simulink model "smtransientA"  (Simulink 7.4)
settings: Solver=ode45  StartTime=0.0  StopTime=5  MaxStep=1e-3  RelTol=1e-4  AbsTol=1e-4
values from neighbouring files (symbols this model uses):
  Bm = 0.10    (= 0.1)    [IMabc2.m]    (also in imabcparam.m = 0.01; IMabcrun0.m = 0.01; IMabcrun1.m = 0.001; IMcur0.m = 1e-06)
  H = 0.60    (= 0.6)    [IMabc2.m]    (also in IMcur0.m = 0.3; imdef0vec.m = 0.3; imdef1vec.m = 0.3; imdef2vec.m = 0.3)
  n0 = 0.98    [imdef0vec.m]    (also in imdef1vec.m = 0.978; imdef2vec.m; imdefrotflux.m; imdefSIvec1.m = 0.95)
  Ra = .95    (= 0.95)    [altwdgs.m]    (also in Ccurverun.m = 0.018)
  tc = abs(fco)    [im3phase.m]
  Te0 = 0.75/wo*p*(Is*conj(Is)*Req)    [imdefSIvec1.m]
  V = [Vas 0 0].'    [Actac.m]    (also in acttrcalc1.m = str2num(get(h,'string')); im3d.m = eval(get(hVs,'String')); IMabc2.m = [vas vbs vcs 0 0 0]'; IMabcf0.m = [vas vbs vcs 0 0 0]')
  wo = 2*pi*freq0    [calc0.m]    (also in IMabc2.m = 376.991118431; imabcparam.m = 376.991118431; IMabcrun0.m = 376.991118431; IMabcrun1.m = 376.991118431)
undefined symbols (not defined in the file or in its folder): delta0, fk0, L_1, phif0, Rf, Rkd, Rkq, vf0

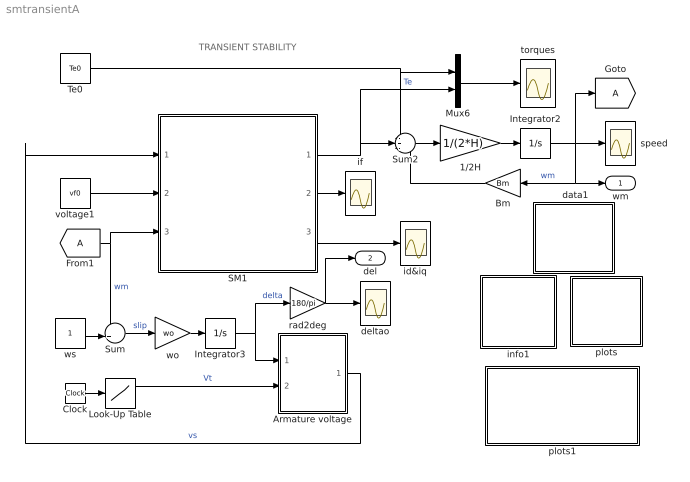
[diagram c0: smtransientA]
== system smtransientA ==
  note: TRANSIENT STABILITY
  " data1" : Subsystem
  1/2H : Gain  Gain=1/(2*H)  ParameterDataType=sfix(16)  ParameterScaling=2^0  OutDataType=sfix(16)  OutScaling=2^0
  Armature voltage : Subsystem
  Bm : Gain  Gain=Bm  ParameterDataType=sfix(16)  ParameterScaling=2^0  OutDataType=sfix(16)  OutScaling=2^0
  Clock : Clock
  Integrator2 : Integrator  InitialCondition=n0
  Integrator3 : Integrator  InitialCondition=delta0
  Look-Up Table : Lookup  InputValues=[0 0.5 0.5 0.5+tc 0.5+tc 3]  Table=[V V 0 0 V V]  OutDataType=sfix(16)  OutScaling=2^0
  Mux6 : Mux  Inputs=2
  SM1 : Subsystem
  Sum : Sum  Inputs=-+|  OutDataType=sfix(16)  OutScaling=2^0
  Sum2 : Sum  Inputs=-+-  OutDataType=sfix(16)  OutScaling=2^0
  Te0 : Constant  Value=Te0  OutDataType=sfix(16)  OutScaling=2^0
  deltao : Scope
  id&iq : Scope
  if : Scope
  info1 : Subsystem
  plots : Subsystem
  plots1 : Subsystem
  rad2deg : Gain  Gain=180/pi  ParameterDataType=sfix(16)  ParameterScaling=2^0  OutDataType=sfix(16)  OutScaling=2^0
  speed : Scope
  torques : Scope
  voltage1 : Constant  Value=vf0  OutDataType=sfix(16)  OutScaling=2^0
  wo : Gain  Gain=wo  ParameterDataType=sfix(16)  ParameterScaling=2^0  OutDataType=sfix(16)  OutScaling=2^0
  ws : Constant  OutDataType=sfix(16)  OutScaling=2^0
  wm : Outport
  del : Outport  Port=2
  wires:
  Mux6/1 -> torques/1
  voltage1/1 -> SM1/2(vf)
  SM1/2(if) -> if/1
  Sum2/1 -> 1/2H/1
  1/2H/1 -> Integrator2/1
  SM1/1(Te) -> Sum2/2, Mux6/2  "Te"
  Bm/1 -> Sum2/3
  Integrator2/1 -> speed/1, [A], Bm/1, wm/1  "wm"
  Te0/1 -> Mux6/1, Sum2/1
  ws/1 -> Sum/2
  Sum/1 -> wo/1  "slip"
  wo/1 -> Integrator3/1
  Armature voltage/1(vs) -> SM1/1(vs)  "vs"
  Integrator3/1 -> Armature voltage/1(delta), rad2deg/1  "delta"
  SM1/3(ia) -> id&iq/1
  rad2deg/1 -> deltao/1, del/1
  Clock/1 -> Look-Up Table/1
  Look-Up Table/1 -> Armature voltage/2(Vt)  "Vt"
  [A] -> Sum/1, SM1/3(wm)  "wm"

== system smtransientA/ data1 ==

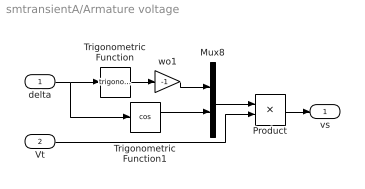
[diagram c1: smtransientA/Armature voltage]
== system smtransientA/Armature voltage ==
  delta : Inport  OutDataType=sfix(16)  OutScaling=2^0
  Vt : Inport  Port=2  OutDataType=sfix(16)  OutScaling=2^0
  Mux8 : Mux  Inputs=2
  Product : Product  OutDataType=sfix(16)  OutScaling=2^0
  Trigonometric Function : Trigonometry
  Trigonometric Function1 : Trigonometry  Operator=cos
  wo1 : Gain  Gain=-1  ParameterDataType=sfix(16)  ParameterScaling=2^0  OutDataType=sfix(16)  OutScaling=2^0
  vs : Outport
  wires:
  delta/1 -> Trigonometric Function/1, Trigonometric Function1/1
  Trigonometric Function/1 -> wo1/1
  Mux8/1 -> Product/1
  wo1/1 -> Mux8/1
  Trigonometric Function1/1 -> Mux8/2
  Product/1 -> vs/1
  Vt/1 -> Product/2

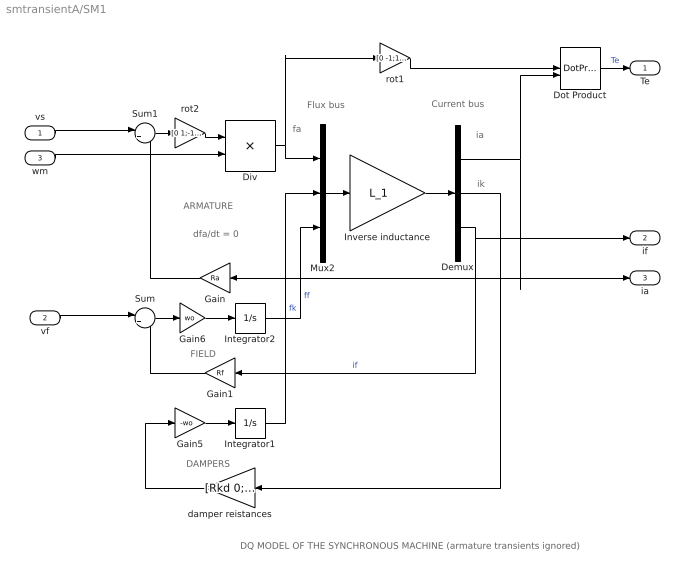
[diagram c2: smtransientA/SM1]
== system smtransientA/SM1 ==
  note: DAMPERS
  note: ARMATURE
  note: fa
  note: ia
  note: FIELD
  note: DQ MODEL OF THE SYNCHRONOUS MACHINE (armature transients ignored)
  note: Flux bus
  note: Current bus
  note: dfa/dt = 0
  note: ik
  vs : Inport  OutDataType=sfix(16)  OutScaling=2^0
  vf : Inport  Port=2  OutDataType=sfix(16)  OutScaling=2^0
  wm : Inport  Port=3  OutDataType=sfix(16)  OutScaling=2^0
  Demux : Demux  Outputs=3
  Div : Product  Inputs=*/  Multiplication=Matrix(*)  OutDataType=sfix(16)  OutScaling=2^0
  Dot Product : DotProduct  OutDataType=fixdt(1, 16)  OutScaling=2^-10
  Gain : Gain  Gain=Ra  ParameterDataType=sfix(16)  ParameterScaling=2^0  OutDataType=sfix(16)  OutScaling=2^0
  Gain1 : Gain  Gain=Rf  ParameterDataType=sfix(16)  ParameterScaling=2^0  OutDataType=sfix(16)  OutScaling=2^0
  Gain5 : Gain  Gain=-wo  ParameterDataType=sfix(16)  ParameterScaling=2^0  OutDataType=sfix(16)  OutScaling=2^0
  Gain6 : Gain  Gain=wo  ParameterDataType=sfix(16)  ParameterScaling=2^0  OutDataType=sfix(16)  OutScaling=2^0
  Integrator1 : Integrator  InitialCondition=fk0
  Integrator2 : Integrator  InitialCondition=phif0
  Inverse inductance : Gain  Gain=L_1  Multiplication=Matrix(K*u)  ParameterDataType=sfix(16)  ParameterScaling=2^0  OutDataType=sfix(16)  OutScaling=2^0
  Mux2 : Mux  Inputs=3
  Sum : Sum  Inputs=|+-  OutDataType=sfix(16)  OutScaling=2^0
  Sum1 : Sum  Inputs=|+-  OutDataType=sfix(16)  OutScaling=2^0
  damper reistances : Gain  Gain=[Rkd 0;0 Rkq]  Multiplication=Matrix(K*u)  ParameterDataType=sfix(16)  ParameterScaling=2^0  OutDataType=sfix(16)  OutScaling=2^0
  rot1 : Gain  Gain=[0 -1;1 0]  Multiplication=Matrix(K*u)  ParameterDataType=sfix(16)  ParameterScaling=2^0  OutDataType=sfix(16)  OutScaling=2^0
  rot2 : Gain  Gain=[0 1;-1 0]  Multiplication=Matrix(K*u)  ParameterDataType=sfix(16)  ParameterScaling=2^0  OutDataType=sfix(16)  OutScaling=2^0
  Te : Outport
  if : Outport  Port=2
  ia : Outport  Port=3
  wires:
  Gain5/1 -> Integrator1/1
  damper reistances/1 -> Gain5/1
  Sum1/1 -> rot2/1
  Gain/1 -> Sum1/2
  Gain6/1 -> Integrator2/1
  Sum/1 -> Gain6/1
  vf/1 -> Sum/1
  Gain1/1 -> Sum/2
  rot1/1 -> Dot Product/1
  Demux/1 -> Gain/1, ia/1, Dot Product/2
  Dot Product/1 -> Te/1  "Te"
  Mux2/1 -> Inverse inductance/1
  Inverse inductance/1 -> Demux/1
  Integrator1/1 -> Mux2/2  "fk"
  Integrator2/1 -> Mux2/3  "ff"
  Demux/2 -> damper reistances/1
  Demux/3 -> if/1, Gain1/1  "if"
  vs/1 -> Sum1/1
  Div/1 -> Mux2/1, rot1/1
  rot2/1 -> Div/1
  wm/1 -> Div/2

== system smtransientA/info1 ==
  note: Synchronous machine transient stability
  note: This demonstration illustrates the dynamics of a synchronous machine following the sudden application and removal of a three-phase short circuit at the terminals. Four models of the synchronous machine are provided: 1) A complete model (5th-order) 2) Armature transients ignored by setting dfa/dt=0 (3rd-order) 3) Both armature transients and damper effects are neglected (1st-order) 4) Constant field flux linkage (zero-order) Click the DATA block to enter the parameters and prefault operating conditions. Initialize and then Start the simulation.

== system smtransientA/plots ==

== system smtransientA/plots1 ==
